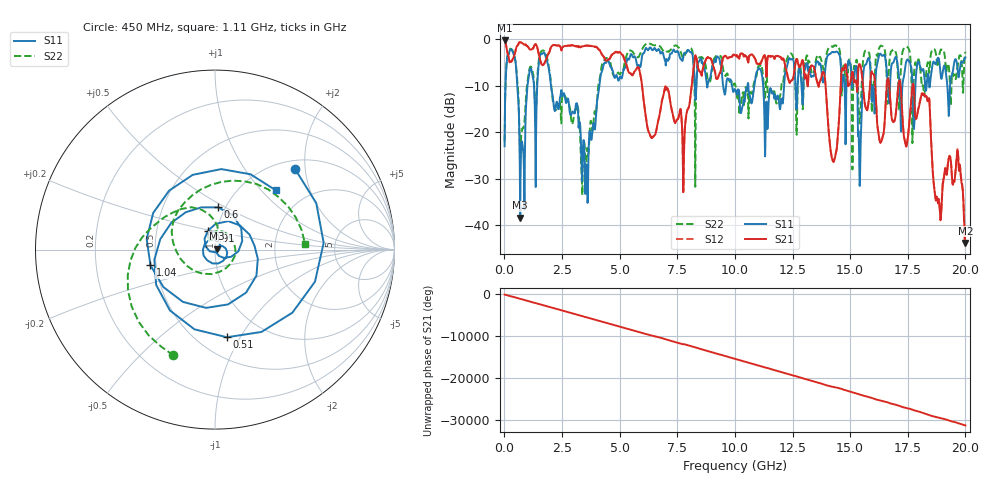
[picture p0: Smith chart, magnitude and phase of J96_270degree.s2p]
!Keysight Technologies,N5222A,MY51421036,A.10.65.16
!Date: Friday, March 31, 2023 14:25:36
!Correction: S11(Full 2 Port(1,2))
!S21(Full 2 Port(1,2))
!S12(Full 2 Port(1,2))
!S22(Full 2 Port(1,2))
!S2P File: Measurements: S11, S21, S12, S22:
# Hz S  dB  R 50
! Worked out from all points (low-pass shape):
!   2000 points, 10 MHz to 20 GHz, reference 50 ohm
!   highest |S21| = -0.24 dB at 10 MHz (marker M1); lowest = -43.9 dB at 20 GHz (marker M2)
!   |S21| within 3 dB of the highest: 439.3 MHz to 1.494 GHz (1.054 GHz wide, 109 % of centre); 1.899 GHz to 4.225 GHz (2.326 GHz wide, 76 % of centre)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
!   lowest |S11| = -38.5 dB at 690 MHz (marker M3), VSWR 1.02, Z = 51 + j0.599 ohm
!   |S11| at or under -10 dB: 2.022 GHz to 4.119 GHz (2.097 GHz wide, 68.3 % of centre); 9.87 GHz to 10.54 GHz (674.7 MHz wide, 6.61 % of centre); 11.23 GHz to 12.13 GHz (906.1 MHz wide, 7.76 % of centre)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
!   |S22| runs from -33.6 to -0.9 dB; largest |S21 - S12| = 0.012
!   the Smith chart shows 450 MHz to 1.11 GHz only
!   S11 on the Smith chart (normalised r, x): 450 MHz: 1.18, +1.77; 510 MHz: 0.68, -0.88; 600 MHz: 0.93, +0.46; 910 MHz: 0.91, +0.19; 1.04 GHz: 0.47, -0.09; 1.11 GHz: 1.42, +1.21
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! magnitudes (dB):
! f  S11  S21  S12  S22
! 10 MHz  -23.0  -0.2  -0.3  -22.0
! 450 MHz  -4.0  -3.1  -3.1  -4.0
! 510 MHz  -6.1  -1.9  -1.9  -5.9
! 600 MHz  -12.5  -1.1  -1.1  -11.4
! 690 MHz  -38.5  -0.6  -0.6  -24.9
! 910 MHz  -18.9  -1.1  -1.1  -14.9
! 1.04 GHz  -8.6  -1.7  -1.7  -7.7
! 1.11 GHz  -6.5  -2.2  -2.2  -6.0
! 3.35 GHz  -28.0  -1.5  -1.5  -30.1
! 4.33 GHz  -5.2  -3.9  -3.8  -4.6
! 6.68 GHz  -2.1  -17.4  -17.4  -1.3
! 10.01 GHz  -10.8  -3.4  -3.5  -9.6
! 13.34 GHz  -8.0  -5.7  -5.6  -7.3
! 14.27 GHz  -2.8  -26.3  -26.3  -1.6
! 14.72 GHz  -7.8  -6.6  -6.5  -5.6
! 15.43 GHz  -28.9  -5.5  -5.5  -17.9
! 16.33 GHz  -3.2  -22.2  -22.2  -1.4
! 16.67 GHz  -12.0  -8.9  -8.8  -7.5
! 18.35 GHz  -8.0  -13.2  -13.1  -5.2
! 18.73 GHz  -5.2  -34.7  -34.4  -3.3
! 19.69 GHz  -7.8  -25.5  -25.2  -5.0
! 20 GHz  -3.9  -43.9  -44.6  -2.7
